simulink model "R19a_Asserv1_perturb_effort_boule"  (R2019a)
settings: Solver=ode15s  StartTime=0.0  StopTime=1  RelTol=1e-3  EnableMultiTasking=on
undefined symbols (not defined in the file): deg, kg, m, manette1_Défaut_sldprt, manette2_Défaut_sldprt, mm, N, rad, s, sigbuilder_block, STL, X, Y, Z
libraries: sm_lib x460, fl_lib x45, nesl_utility x23, simulink x3
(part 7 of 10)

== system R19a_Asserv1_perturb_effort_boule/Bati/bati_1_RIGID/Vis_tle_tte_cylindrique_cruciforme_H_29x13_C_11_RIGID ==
  ReferenceFrame : sm_lib/Frames and Transforms/Reference Frame
  Solid : sm_lib/Body Elements/Solid  InertiaType=Custom  Mass=8.3821869835456372e-05  MassUnits=kg  CenterOfMass=[4.9478681581074904 0.00064910481891303923 -0.0013634218224953438]  CenterOfMassUnits=mm  MomentsOfInertia=[0.00016543197172893975 0.0014334630955093895 0.0014333390308476422]  MomentsOfInertiaUnits=kg*mm^2  ProductsOfInertia=[-5.4062904633677868e-09 -1.3111174919527308e-07 6.0713893531177014e-07]  ProductsOfInertiaUnits=kg*mm^2  BasedOnType=Density  Density=1000  DensityUnits=kg/(m^3)  DoExposeReferenceFrame=on  SerializedFrames=<Frames/>  GraphicType=FromGeometry  MarkerShape=Sphere  MarkerSize=10  MarkerSizeUnits=m  GraphicVisPropType=SimpleVisualProperties  GraphicDiffuseColor=[0.75294117647058822 0.75294117647058822 0.75294117647058822]  GraphicSpecularColor=[0.5 0.5 0.5 1.0]  GraphicAmbientColor=[0.15 0.15 0.15 1.0]  GraphicEmissiveColor=[0.0 0.0 0.0 1.0]  GraphicShininess=75  GraphicOpacity=1  GeometryShape=FromFile  RectangleSize=[1 1]  RectangleSizeUnits=m  BrickDimensions=[1 1 1]  BrickDimensionUnits=m  CylinderRadius=1  CylinderRadiusUnits=m  CylinderLength=1  CylinderLengthUnits=m  SphereRadius=1  SphereRadiusUnits=m  EllipsoidRadii=[1 1 1]  EllipsoidRadiiUnits=m  ExtrusionCrossSection=[1 1; -1 1; -1 -1; 1 -1]  ExtrusionCrossSectionUnits=m  ExtrusionLength=1  ExtrusionLengthUnits=m  PolygonNumSides=3  PolygonOuterRadius=1  PolygonOuterRadiusUnits=m  ExtGeomFileType=STL  ExtGeomFileName=\STL\Vis à tôle tête cylindrique cruciforme H 2-9x13 - C_Réaliste_sldprt.STL  ExtGeomFileUnits=mm  RevolutionCrossSection=[1 1; 1 -1; 2 -1; 2 1]  RevolutionCrossSectionUnits=m  RevolutionExtent=Full  RevolutionAngle=180  RevolutionAngleUnits=deg
  F : PMIOPort  Side=Left
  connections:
  Solid/RConn1 -- ReferenceFrame/RConn1 -- F/RConn1

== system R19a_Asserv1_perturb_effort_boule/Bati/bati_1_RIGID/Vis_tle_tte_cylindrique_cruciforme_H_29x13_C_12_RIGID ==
  ReferenceFrame : sm_lib/Frames and Transforms/Reference Frame
  Solid : sm_lib/Body Elements/Solid  InertiaType=Custom  Mass=8.3821869835456372e-05  MassUnits=kg  CenterOfMass=[4.9478681581074904 0.00064910481891303923 -0.0013634218224953438]  CenterOfMassUnits=mm  MomentsOfInertia=[0.00016543197172893975 0.0014334630955093895 0.0014333390308476422]  MomentsOfInertiaUnits=kg*mm^2  ProductsOfInertia=[-5.4062904633677868e-09 -1.3111174919527308e-07 6.0713893531177014e-07]  ProductsOfInertiaUnits=kg*mm^2  BasedOnType=Density  Density=1000  DensityUnits=kg/(m^3)  DoExposeReferenceFrame=on  SerializedFrames=<Frames/>  GraphicType=FromGeometry  MarkerShape=Sphere  MarkerSize=10  MarkerSizeUnits=m  GraphicVisPropType=SimpleVisualProperties  GraphicDiffuseColor=[0.75294117647058822 0.75294117647058822 0.75294117647058822]  GraphicSpecularColor=[0.5 0.5 0.5 1.0]  GraphicAmbientColor=[0.15 0.15 0.15 1.0]  GraphicEmissiveColor=[0.0 0.0 0.0 1.0]  GraphicShininess=75  GraphicOpacity=1  GeometryShape=FromFile  RectangleSize=[1 1]  RectangleSizeUnits=m  BrickDimensions=[1 1 1]  BrickDimensionUnits=m  CylinderRadius=1  CylinderRadiusUnits=m  CylinderLength=1  CylinderLengthUnits=m  SphereRadius=1  SphereRadiusUnits=m  EllipsoidRadii=[1 1 1]  EllipsoidRadiiUnits=m  ExtrusionCrossSection=[1 1; -1 1; -1 -1; 1 -1]  ExtrusionCrossSectionUnits=m  ExtrusionLength=1  ExtrusionLengthUnits=m  PolygonNumSides=3  PolygonOuterRadius=1  PolygonOuterRadiusUnits=m  ExtGeomFileType=STL  ExtGeomFileName=\STL\Vis à tôle tête cylindrique cruciforme H 2-9x13 - C_Réaliste_sldprt.STL  ExtGeomFileUnits=mm  RevolutionCrossSection=[1 1; 1 -1; 2 -1; 2 1]  RevolutionCrossSectionUnits=m  RevolutionExtent=Full  RevolutionAngle=180  RevolutionAngleUnits=deg
  F : PMIOPort  Side=Left
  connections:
  Solid/RConn1 -- ReferenceFrame/RConn1 -- F/RConn1

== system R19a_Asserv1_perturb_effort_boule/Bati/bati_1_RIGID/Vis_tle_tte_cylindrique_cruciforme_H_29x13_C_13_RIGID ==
  ReferenceFrame : sm_lib/Frames and Transforms/Reference Frame
  Solid : sm_lib/Body Elements/Solid  InertiaType=Custom  Mass=8.3821869835456372e-05  MassUnits=kg  CenterOfMass=[4.9478681581074904 0.00064910481891303923 -0.0013634218224953438]  CenterOfMassUnits=mm  MomentsOfInertia=[0.00016543197172893975 0.0014334630955093895 0.0014333390308476422]  MomentsOfInertiaUnits=kg*mm^2  ProductsOfInertia=[-5.4062904633677868e-09 -1.3111174919527308e-07 6.0713893531177014e-07]  ProductsOfInertiaUnits=kg*mm^2  BasedOnType=Density  Density=1000  DensityUnits=kg/(m^3)  DoExposeReferenceFrame=on  SerializedFrames=<Frames/>  GraphicType=FromGeometry  MarkerShape=Sphere  MarkerSize=10  MarkerSizeUnits=m  GraphicVisPropType=SimpleVisualProperties  GraphicDiffuseColor=[0.75294117647058822 0.75294117647058822 0.75294117647058822]  GraphicSpecularColor=[0.5 0.5 0.5 1.0]  GraphicAmbientColor=[0.15 0.15 0.15 1.0]  GraphicEmissiveColor=[0.0 0.0 0.0 1.0]  GraphicShininess=75  GraphicOpacity=1  GeometryShape=FromFile  RectangleSize=[1 1]  RectangleSizeUnits=m  BrickDimensions=[1 1 1]  BrickDimensionUnits=m  CylinderRadius=1  CylinderRadiusUnits=m  CylinderLength=1  CylinderLengthUnits=m  SphereRadius=1  SphereRadiusUnits=m  EllipsoidRadii=[1 1 1]  EllipsoidRadiiUnits=m  ExtrusionCrossSection=[1 1; -1 1; -1 -1; 1 -1]  ExtrusionCrossSectionUnits=m  ExtrusionLength=1  ExtrusionLengthUnits=m  PolygonNumSides=3  PolygonOuterRadius=1  PolygonOuterRadiusUnits=m  ExtGeomFileType=STL  ExtGeomFileName=\STL\Vis à tôle tête cylindrique cruciforme H 2-9x13 - C_Réaliste_sldprt.STL  ExtGeomFileUnits=mm  RevolutionCrossSection=[1 1; 1 -1; 2 -1; 2 1]  RevolutionCrossSectionUnits=m  RevolutionExtent=Full  RevolutionAngle=180  RevolutionAngleUnits=deg
  F : PMIOPort  Side=Left
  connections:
  Solid/RConn1 -- ReferenceFrame/RConn1 -- F/RConn1

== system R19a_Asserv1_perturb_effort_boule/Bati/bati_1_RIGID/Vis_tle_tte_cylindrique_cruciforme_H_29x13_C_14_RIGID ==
  ReferenceFrame : sm_lib/Frames and Transforms/Reference Frame
  Solid : sm_lib/Body Elements/Solid  InertiaType=Custom  Mass=8.3821869835456372e-05  MassUnits=kg  CenterOfMass=[4.9478681581074904 0.00064910481891303923 -0.0013634218224953438]  CenterOfMassUnits=mm  MomentsOfInertia=[0.00016543197172893975 0.0014334630955093895 0.0014333390308476422]  MomentsOfInertiaUnits=kg*mm^2  ProductsOfInertia=[-5.4062904633677868e-09 -1.3111174919527308e-07 6.0713893531177014e-07]  ProductsOfInertiaUnits=kg*mm^2  BasedOnType=Density  Density=1000  DensityUnits=kg/(m^3)  DoExposeReferenceFrame=on  SerializedFrames=<Frames/>  GraphicType=FromGeometry  MarkerShape=Sphere  MarkerSize=10  MarkerSizeUnits=m  GraphicVisPropType=SimpleVisualProperties  GraphicDiffuseColor=[0.75294117647058822 0.75294117647058822 0.75294117647058822]  GraphicSpecularColor=[0.5 0.5 0.5 1.0]  GraphicAmbientColor=[0.15 0.15 0.15 1.0]  GraphicEmissiveColor=[0.0 0.0 0.0 1.0]  GraphicShininess=75  GraphicOpacity=1  GeometryShape=FromFile  RectangleSize=[1 1]  RectangleSizeUnits=m  BrickDimensions=[1 1 1]  BrickDimensionUnits=m  CylinderRadius=1  CylinderRadiusUnits=m  CylinderLength=1  CylinderLengthUnits=m  SphereRadius=1  SphereRadiusUnits=m  EllipsoidRadii=[1 1 1]  EllipsoidRadiiUnits=m  ExtrusionCrossSection=[1 1; -1 1; -1 -1; 1 -1]  ExtrusionCrossSectionUnits=m  ExtrusionLength=1  ExtrusionLengthUnits=m  PolygonNumSides=3  PolygonOuterRadius=1  PolygonOuterRadiusUnits=m  ExtGeomFileType=STL  ExtGeomFileName=\STL\Vis à tôle tête cylindrique cruciforme H 2-9x13 - C_Réaliste_sldprt.STL  ExtGeomFileUnits=mm  RevolutionCrossSection=[1 1; 1 -1; 2 -1; 2 1]  RevolutionCrossSectionUnits=m  RevolutionExtent=Full  RevolutionAngle=180  RevolutionAngleUnits=deg
  F : PMIOPort  Side=Left
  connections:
  Solid/RConn1 -- ReferenceFrame/RConn1 -- F/RConn1

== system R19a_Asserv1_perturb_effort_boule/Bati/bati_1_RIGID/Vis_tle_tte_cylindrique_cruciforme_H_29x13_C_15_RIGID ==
  ReferenceFrame : sm_lib/Frames and Transforms/Reference Frame
  Solid : sm_lib/Body Elements/Solid  InertiaType=Custom  Mass=8.3821869835456372e-05  MassUnits=kg  CenterOfMass=[4.9478681581074904 0.00064910481891303923 -0.0013634218224953438]  CenterOfMassUnits=mm  MomentsOfInertia=[0.00016543197172893975 0.0014334630955093895 0.0014333390308476422]  MomentsOfInertiaUnits=kg*mm^2  ProductsOfInertia=[-5.4062904633677868e-09 -1.3111174919527308e-07 6.0713893531177014e-07]  ProductsOfInertiaUnits=kg*mm^2  BasedOnType=Density  Density=1000  DensityUnits=kg/(m^3)  DoExposeReferenceFrame=on  SerializedFrames=<Frames/>  GraphicType=FromGeometry  MarkerShape=Sphere  MarkerSize=10  MarkerSizeUnits=m  GraphicVisPropType=SimpleVisualProperties  GraphicDiffuseColor=[0.75294117647058822 0.75294117647058822 0.75294117647058822]  GraphicSpecularColor=[0.5 0.5 0.5 1.0]  GraphicAmbientColor=[0.15 0.15 0.15 1.0]  GraphicEmissiveColor=[0.0 0.0 0.0 1.0]  GraphicShininess=75  GraphicOpacity=1  GeometryShape=FromFile  RectangleSize=[1 1]  RectangleSizeUnits=m  BrickDimensions=[1 1 1]  BrickDimensionUnits=m  CylinderRadius=1  CylinderRadiusUnits=m  CylinderLength=1  CylinderLengthUnits=m  SphereRadius=1  SphereRadiusUnits=m  EllipsoidRadii=[1 1 1]  EllipsoidRadiiUnits=m  ExtrusionCrossSection=[1 1; -1 1; -1 -1; 1 -1]  ExtrusionCrossSectionUnits=m  ExtrusionLength=1  ExtrusionLengthUnits=m  PolygonNumSides=3  PolygonOuterRadius=1  PolygonOuterRadiusUnits=m  ExtGeomFileType=STL  ExtGeomFileName=\STL\Vis à tôle tête cylindrique cruciforme H 2-9x13 - C_Réaliste_sldprt.STL  ExtGeomFileUnits=mm  RevolutionCrossSection=[1 1; 1 -1; 2 -1; 2 1]  RevolutionCrossSectionUnits=m  RevolutionExtent=Full  RevolutionAngle=180  RevolutionAngleUnits=deg
  F : PMIOPort  Side=Left
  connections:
  Solid/RConn1 -- ReferenceFrame/RConn1 -- F/RConn1

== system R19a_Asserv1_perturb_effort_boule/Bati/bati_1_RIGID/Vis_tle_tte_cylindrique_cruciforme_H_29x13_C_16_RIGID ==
  ReferenceFrame : sm_lib/Frames and Transforms/Reference Frame
  Solid : sm_lib/Body Elements/Solid  InertiaType=Custom  Mass=8.3821869835456372e-05  MassUnits=kg  CenterOfMass=[4.9478681581074904 0.00064910481891303923 -0.0013634218224953438]  CenterOfMassUnits=mm  MomentsOfInertia=[0.00016543197172893975 0.0014334630955093895 0.0014333390308476422]  MomentsOfInertiaUnits=kg*mm^2  ProductsOfInertia=[-5.4062904633677868e-09 -1.3111174919527308e-07 6.0713893531177014e-07]  ProductsOfInertiaUnits=kg*mm^2  BasedOnType=Density  Density=1000  DensityUnits=kg/(m^3)  DoExposeReferenceFrame=on  SerializedFrames=<Frames/>  GraphicType=FromGeometry  MarkerShape=Sphere  MarkerSize=10  MarkerSizeUnits=m  GraphicVisPropType=SimpleVisualProperties  GraphicDiffuseColor=[0.75294117647058822 0.75294117647058822 0.75294117647058822]  GraphicSpecularColor=[0.5 0.5 0.5 1.0]  GraphicAmbientColor=[0.15 0.15 0.15 1.0]  GraphicEmissiveColor=[0.0 0.0 0.0 1.0]  GraphicShininess=75  GraphicOpacity=1  GeometryShape=FromFile  RectangleSize=[1 1]  RectangleSizeUnits=m  BrickDimensions=[1 1 1]  BrickDimensionUnits=m  CylinderRadius=1  CylinderRadiusUnits=m  CylinderLength=1  CylinderLengthUnits=m  SphereRadius=1  SphereRadiusUnits=m  EllipsoidRadii=[1 1 1]  EllipsoidRadiiUnits=m  ExtrusionCrossSection=[1 1; -1 1; -1 -1; 1 -1]  ExtrusionCrossSectionUnits=m  ExtrusionLength=1  ExtrusionLengthUnits=m  PolygonNumSides=3  PolygonOuterRadius=1  PolygonOuterRadiusUnits=m  ExtGeomFileType=STL  ExtGeomFileName=\STL\Vis à tôle tête cylindrique cruciforme H 2-9x13 - C_Réaliste_sldprt.STL  ExtGeomFileUnits=mm  RevolutionCrossSection=[1 1; 1 -1; 2 -1; 2 1]  RevolutionCrossSectionUnits=m  RevolutionExtent=Full  RevolutionAngle=180  RevolutionAngleUnits=deg
  F : PMIOPort  Side=Left
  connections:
  Solid/RConn1 -- ReferenceFrame/RConn1 -- F/RConn1

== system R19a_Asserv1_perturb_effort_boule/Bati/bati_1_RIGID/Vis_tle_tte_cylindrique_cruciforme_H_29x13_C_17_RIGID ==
  ReferenceFrame : sm_lib/Frames and Transforms/Reference Frame
  Solid : sm_lib/Body Elements/Solid  InertiaType=Custom  Mass=8.3821869835456372e-05  MassUnits=kg  CenterOfMass=[4.9478681581074904 0.00064910481891303923 -0.0013634218224953438]  CenterOfMassUnits=mm  MomentsOfInertia=[0.00016543197172893975 0.0014334630955093895 0.0014333390308476422]  MomentsOfInertiaUnits=kg*mm^2  ProductsOfInertia=[-5.4062904633677868e-09 -1.3111174919527308e-07 6.0713893531177014e-07]  ProductsOfInertiaUnits=kg*mm^2  BasedOnType=Density  Density=1000  DensityUnits=kg/(m^3)  DoExposeReferenceFrame=on  SerializedFrames=<Frames/>  GraphicType=FromGeometry  MarkerShape=Sphere  MarkerSize=10  MarkerSizeUnits=m  GraphicVisPropType=SimpleVisualProperties  GraphicDiffuseColor=[0.75294117647058822 0.75294117647058822 0.75294117647058822]  GraphicSpecularColor=[0.5 0.5 0.5 1.0]  GraphicAmbientColor=[0.15 0.15 0.15 1.0]  GraphicEmissiveColor=[0.0 0.0 0.0 1.0]  GraphicShininess=75  GraphicOpacity=1  GeometryShape=FromFile  RectangleSize=[1 1]  RectangleSizeUnits=m  BrickDimensions=[1 1 1]  BrickDimensionUnits=m  CylinderRadius=1  CylinderRadiusUnits=m  CylinderLength=1  CylinderLengthUnits=m  SphereRadius=1  SphereRadiusUnits=m  EllipsoidRadii=[1 1 1]  EllipsoidRadiiUnits=m  ExtrusionCrossSection=[1 1; -1 1; -1 -1; 1 -1]  ExtrusionCrossSectionUnits=m  ExtrusionLength=1  ExtrusionLengthUnits=m  PolygonNumSides=3  PolygonOuterRadius=1  PolygonOuterRadiusUnits=m  ExtGeomFileType=STL  ExtGeomFileName=\STL\Vis à tôle tête cylindrique cruciforme H 2-9x13 - C_Réaliste_sldprt.STL  ExtGeomFileUnits=mm  RevolutionCrossSection=[1 1; 1 -1; 2 -1; 2 1]  RevolutionCrossSectionUnits=m  RevolutionExtent=Full  RevolutionAngle=180  RevolutionAngleUnits=deg
  F : PMIOPort  Side=Left
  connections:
  Solid/RConn1 -- ReferenceFrame/RConn1 -- F/RConn1

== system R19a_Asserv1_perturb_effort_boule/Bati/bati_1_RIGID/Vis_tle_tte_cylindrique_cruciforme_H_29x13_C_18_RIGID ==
  ReferenceFrame : sm_lib/Frames and Transforms/Reference Frame
  Solid : sm_lib/Body Elements/Solid  InertiaType=Custom  Mass=8.3821869835456372e-05  MassUnits=kg  CenterOfMass=[4.9478681581074904 0.00064910481891303923 -0.0013634218224953438]  CenterOfMassUnits=mm  MomentsOfInertia=[0.00016543197172893975 0.0014334630955093895 0.0014333390308476422]  MomentsOfInertiaUnits=kg*mm^2  ProductsOfInertia=[-5.4062904633677868e-09 -1.3111174919527308e-07 6.0713893531177014e-07]  ProductsOfInertiaUnits=kg*mm^2  BasedOnType=Density  Density=1000  DensityUnits=kg/(m^3)  DoExposeReferenceFrame=on  SerializedFrames=<Frames/>  GraphicType=FromGeometry  MarkerShape=Sphere  MarkerSize=10  MarkerSizeUnits=m  GraphicVisPropType=SimpleVisualProperties  GraphicDiffuseColor=[0.75294117647058822 0.75294117647058822 0.75294117647058822]  GraphicSpecularColor=[0.5 0.5 0.5 1.0]  GraphicAmbientColor=[0.15 0.15 0.15 1.0]  GraphicEmissiveColor=[0.0 0.0 0.0 1.0]  GraphicShininess=75  GraphicOpacity=1  GeometryShape=FromFile  RectangleSize=[1 1]  RectangleSizeUnits=m  BrickDimensions=[1 1 1]  BrickDimensionUnits=m  CylinderRadius=1  CylinderRadiusUnits=m  CylinderLength=1  CylinderLengthUnits=m  SphereRadius=1  SphereRadiusUnits=m  EllipsoidRadii=[1 1 1]  EllipsoidRadiiUnits=m  ExtrusionCrossSection=[1 1; -1 1; -1 -1; 1 -1]  ExtrusionCrossSectionUnits=m  ExtrusionLength=1  ExtrusionLengthUnits=m  PolygonNumSides=3  PolygonOuterRadius=1  PolygonOuterRadiusUnits=m  ExtGeomFileType=STL  ExtGeomFileName=\STL\Vis à tôle tête cylindrique cruciforme H 2-9x13 - C_Réaliste_sldprt.STL  ExtGeomFileUnits=mm  RevolutionCrossSection=[1 1; 1 -1; 2 -1; 2 1]  RevolutionCrossSectionUnits=m  RevolutionExtent=Full  RevolutionAngle=180  RevolutionAngleUnits=deg
  F : PMIOPort  Side=Left
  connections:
  Solid/RConn1 -- ReferenceFrame/RConn1 -- F/RConn1

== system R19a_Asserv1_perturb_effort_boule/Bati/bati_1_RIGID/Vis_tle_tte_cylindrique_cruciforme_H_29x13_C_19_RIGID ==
  ReferenceFrame : sm_lib/Frames and Transforms/Reference Frame
  Solid : sm_lib/Body Elements/Solid  InertiaType=Custom  Mass=8.3821869835456372e-05  MassUnits=kg  CenterOfMass=[4.9478681581074904 0.00064910481891303923 -0.0013634218224953438]  CenterOfMassUnits=mm  MomentsOfInertia=[0.00016543197172893975 0.0014334630955093895 0.0014333390308476422]  MomentsOfInertiaUnits=kg*mm^2  ProductsOfInertia=[-5.4062904633677868e-09 -1.3111174919527308e-07 6.0713893531177014e-07]  ProductsOfInertiaUnits=kg*mm^2  BasedOnType=Density  Density=1000  DensityUnits=kg/(m^3)  DoExposeReferenceFrame=on  SerializedFrames=<Frames/>  GraphicType=FromGeometry  MarkerShape=Sphere  MarkerSize=10  MarkerSizeUnits=m  GraphicVisPropType=SimpleVisualProperties  GraphicDiffuseColor=[0.75294117647058822 0.75294117647058822 0.75294117647058822]  GraphicSpecularColor=[0.5 0.5 0.5 1.0]  GraphicAmbientColor=[0.15 0.15 0.15 1.0]  GraphicEmissiveColor=[0.0 0.0 0.0 1.0]  GraphicShininess=75  GraphicOpacity=1  GeometryShape=FromFile  RectangleSize=[1 1]  RectangleSizeUnits=m  BrickDimensions=[1 1 1]  BrickDimensionUnits=m  CylinderRadius=1  CylinderRadiusUnits=m  CylinderLength=1  CylinderLengthUnits=m  SphereRadius=1  SphereRadiusUnits=m  EllipsoidRadii=[1 1 1]  EllipsoidRadiiUnits=m  ExtrusionCrossSection=[1 1; -1 1; -1 -1; 1 -1]  ExtrusionCrossSectionUnits=m  ExtrusionLength=1  ExtrusionLengthUnits=m  PolygonNumSides=3  PolygonOuterRadius=1  PolygonOuterRadiusUnits=m  ExtGeomFileType=STL  ExtGeomFileName=\STL\Vis à tôle tête cylindrique cruciforme H 2-9x13 - C_Réaliste_sldprt.STL  ExtGeomFileUnits=mm  RevolutionCrossSection=[1 1; 1 -1; 2 -1; 2 1]  RevolutionCrossSectionUnits=m  RevolutionExtent=Full  RevolutionAngle=180  RevolutionAngleUnits=deg
  F : PMIOPort  Side=Left
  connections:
  Solid/RConn1 -- ReferenceFrame/RConn1 -- F/RConn1

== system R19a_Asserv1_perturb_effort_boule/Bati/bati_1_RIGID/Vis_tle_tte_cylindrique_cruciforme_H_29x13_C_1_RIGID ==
  ReferenceFrame : sm_lib/Frames and Transforms/Reference Frame
  Solid : sm_lib/Body Elements/Solid  InertiaType=Custom  Mass=8.3821869835456372e-05  MassUnits=kg  CenterOfMass=[4.9478681581074904 0.00064910481891303923 -0.0013634218224953438]  CenterOfMassUnits=mm  MomentsOfInertia=[0.00016543197172893975 0.0014334630955093895 0.0014333390308476422]  MomentsOfInertiaUnits=kg*mm^2  ProductsOfInertia=[-5.4062904633677868e-09 -1.3111174919527308e-07 6.0713893531177014e-07]  ProductsOfInertiaUnits=kg*mm^2  BasedOnType=Density  Density=1000  DensityUnits=kg/(m^3)  DoExposeReferenceFrame=on  SerializedFrames=<Frames/>  GraphicType=FromGeometry  MarkerShape=Sphere  MarkerSize=10  MarkerSizeUnits=m  GraphicVisPropType=SimpleVisualProperties  GraphicDiffuseColor=[0.75294117647058822 0.75294117647058822 0.75294117647058822]  GraphicSpecularColor=[0.5 0.5 0.5 1.0]  GraphicAmbientColor=[0.15 0.15 0.15 1.0]  GraphicEmissiveColor=[0.0 0.0 0.0 1.0]  GraphicShininess=75  GraphicOpacity=1  GeometryShape=FromFile  RectangleSize=[1 1]  RectangleSizeUnits=m  BrickDimensions=[1 1 1]  BrickDimensionUnits=m  CylinderRadius=1  CylinderRadiusUnits=m  CylinderLength=1  CylinderLengthUnits=m  SphereRadius=1  SphereRadiusUnits=m  EllipsoidRadii=[1 1 1]  EllipsoidRadiiUnits=m  ExtrusionCrossSection=[1 1; -1 1; -1 -1; 1 -1]  ExtrusionCrossSectionUnits=m  ExtrusionLength=1  ExtrusionLengthUnits=m  PolygonNumSides=3  PolygonOuterRadius=1  PolygonOuterRadiusUnits=m  ExtGeomFileType=STL  ExtGeomFileName=\STL\Vis à tôle tête cylindrique cruciforme H 2-9x13 - C_Réaliste_sldprt.STL  ExtGeomFileUnits=mm  RevolutionCrossSection=[1 1; 1 -1; 2 -1; 2 1]  RevolutionCrossSectionUnits=m  RevolutionExtent=Full  RevolutionAngle=180  RevolutionAngleUnits=deg
  F : PMIOPort  Side=Left
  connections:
  Solid/RConn1 -- ReferenceFrame/RConn1 -- F/RConn1

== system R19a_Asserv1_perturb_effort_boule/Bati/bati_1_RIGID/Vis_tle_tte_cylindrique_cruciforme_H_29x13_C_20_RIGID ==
  ReferenceFrame : sm_lib/Frames and Transforms/Reference Frame
  Solid : sm_lib/Body Elements/Solid  InertiaType=Custom  Mass=8.3821869835456372e-05  MassUnits=kg  CenterOfMass=[4.9478681581074904 0.00064910481891303923 -0.0013634218224953438]  CenterOfMassUnits=mm  MomentsOfInertia=[0.00016543197172893975 0.0014334630955093895 0.0014333390308476422]  MomentsOfInertiaUnits=kg*mm^2  ProductsOfInertia=[-5.4062904633677868e-09 -1.3111174919527308e-07 6.0713893531177014e-07]  ProductsOfInertiaUnits=kg*mm^2  BasedOnType=Density  Density=1000  DensityUnits=kg/(m^3)  DoExposeReferenceFrame=on  SerializedFrames=<Frames/>  GraphicType=FromGeometry  MarkerShape=Sphere  MarkerSize=10  MarkerSizeUnits=m  GraphicVisPropType=SimpleVisualProperties  GraphicDiffuseColor=[0.75294117647058822 0.75294117647058822 0.75294117647058822]  GraphicSpecularColor=[0.5 0.5 0.5 1.0]  GraphicAmbientColor=[0.15 0.15 0.15 1.0]  GraphicEmissiveColor=[0.0 0.0 0.0 1.0]  GraphicShininess=75  GraphicOpacity=1  GeometryShape=FromFile  RectangleSize=[1 1]  RectangleSizeUnits=m  BrickDimensions=[1 1 1]  BrickDimensionUnits=m  CylinderRadius=1  CylinderRadiusUnits=m  CylinderLength=1  CylinderLengthUnits=m  SphereRadius=1  SphereRadiusUnits=m  EllipsoidRadii=[1 1 1]  EllipsoidRadiiUnits=m  ExtrusionCrossSection=[1 1; -1 1; -1 -1; 1 -1]  ExtrusionCrossSectionUnits=m  ExtrusionLength=1  ExtrusionLengthUnits=m  PolygonNumSides=3  PolygonOuterRadius=1  PolygonOuterRadiusUnits=m  ExtGeomFileType=STL  ExtGeomFileName=\STL\Vis à tôle tête cylindrique cruciforme H 2-9x13 - C_Réaliste_sldprt.STL  ExtGeomFileUnits=mm  RevolutionCrossSection=[1 1; 1 -1; 2 -1; 2 1]  RevolutionCrossSectionUnits=m  RevolutionExtent=Full  RevolutionAngle=180  RevolutionAngleUnits=deg
  F : PMIOPort  Side=Left
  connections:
  Solid/RConn1 -- ReferenceFrame/RConn1 -- F/RConn1

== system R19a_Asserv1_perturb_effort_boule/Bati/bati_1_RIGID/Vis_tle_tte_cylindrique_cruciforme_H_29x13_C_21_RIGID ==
  ReferenceFrame : sm_lib/Frames and Transforms/Reference Frame
  Solid : sm_lib/Body Elements/Solid  InertiaType=Custom  Mass=8.3821869835456372e-05  MassUnits=kg  CenterOfMass=[4.9478681581074904 0.00064910481891303923 -0.0013634218224953438]  CenterOfMassUnits=mm  MomentsOfInertia=[0.00016543197172893975 0.0014334630955093895 0.0014333390308476422]  MomentsOfInertiaUnits=kg*mm^2  ProductsOfInertia=[-5.4062904633677868e-09 -1.3111174919527308e-07 6.0713893531177014e-07]  ProductsOfInertiaUnits=kg*mm^2  BasedOnType=Density  Density=1000  DensityUnits=kg/(m^3)  DoExposeReferenceFrame=on  SerializedFrames=<Frames/>  GraphicType=FromGeometry  MarkerShape=Sphere  MarkerSize=10  MarkerSizeUnits=m  GraphicVisPropType=SimpleVisualProperties  GraphicDiffuseColor=[0.75294117647058822 0.75294117647058822 0.75294117647058822]  GraphicSpecularColor=[0.5 0.5 0.5 1.0]  GraphicAmbientColor=[0.15 0.15 0.15 1.0]  GraphicEmissiveColor=[0.0 0.0 0.0 1.0]  GraphicShininess=75  GraphicOpacity=1  GeometryShape=FromFile  RectangleSize=[1 1]  RectangleSizeUnits=m  BrickDimensions=[1 1 1]  BrickDimensionUnits=m  CylinderRadius=1  CylinderRadiusUnits=m  CylinderLength=1  CylinderLengthUnits=m  SphereRadius=1  SphereRadiusUnits=m  EllipsoidRadii=[1 1 1]  EllipsoidRadiiUnits=m  ExtrusionCrossSection=[1 1; -1 1; -1 -1; 1 -1]  ExtrusionCrossSectionUnits=m  ExtrusionLength=1  ExtrusionLengthUnits=m  PolygonNumSides=3  PolygonOuterRadius=1  PolygonOuterRadiusUnits=m  ExtGeomFileType=STL  ExtGeomFileName=\STL\Vis à tôle tête cylindrique cruciforme H 2-9x13 - C_Réaliste_sldprt.STL  ExtGeomFileUnits=mm  RevolutionCrossSection=[1 1; 1 -1; 2 -1; 2 1]  RevolutionCrossSectionUnits=m  RevolutionExtent=Full  RevolutionAngle=180  RevolutionAngleUnits=deg
  F : PMIOPort  Side=Left
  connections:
  Solid/RConn1 -- ReferenceFrame/RConn1 -- F/RConn1

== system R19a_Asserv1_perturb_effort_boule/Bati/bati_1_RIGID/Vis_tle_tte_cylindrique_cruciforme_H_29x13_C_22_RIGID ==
  ReferenceFrame : sm_lib/Frames and Transforms/Reference Frame
  Solid : sm_lib/Body Elements/Solid  InertiaType=Custom  Mass=8.3821869835456372e-05  MassUnits=kg  CenterOfMass=[4.9478681581074904 0.00064910481891303923 -0.0013634218224953438]  CenterOfMassUnits=mm  MomentsOfInertia=[0.00016543197172893975 0.0014334630955093895 0.0014333390308476422]  MomentsOfInertiaUnits=kg*mm^2  ProductsOfInertia=[-5.4062904633677868e-09 -1.3111174919527308e-07 6.0713893531177014e-07]  ProductsOfInertiaUnits=kg*mm^2  BasedOnType=Density  Density=1000  DensityUnits=kg/(m^3)  DoExposeReferenceFrame=on  SerializedFrames=<Frames/>  GraphicType=FromGeometry  MarkerShape=Sphere  MarkerSize=10  MarkerSizeUnits=m  GraphicVisPropType=SimpleVisualProperties  GraphicDiffuseColor=[0.75294117647058822 0.75294117647058822 0.75294117647058822]  GraphicSpecularColor=[0.5 0.5 0.5 1.0]  GraphicAmbientColor=[0.15 0.15 0.15 1.0]  GraphicEmissiveColor=[0.0 0.0 0.0 1.0]  GraphicShininess=75  GraphicOpacity=1  GeometryShape=FromFile  RectangleSize=[1 1]  RectangleSizeUnits=m  BrickDimensions=[1 1 1]  BrickDimensionUnits=m  CylinderRadius=1  CylinderRadiusUnits=m  CylinderLength=1  CylinderLengthUnits=m  SphereRadius=1  SphereRadiusUnits=m  EllipsoidRadii=[1 1 1]  EllipsoidRadiiUnits=m  ExtrusionCrossSection=[1 1; -1 1; -1 -1; 1 -1]  ExtrusionCrossSectionUnits=m  ExtrusionLength=1  ExtrusionLengthUnits=m  PolygonNumSides=3  PolygonOuterRadius=1  PolygonOuterRadiusUnits=m  ExtGeomFileType=STL  ExtGeomFileName=\STL\Vis à tôle tête cylindrique cruciforme H 2-9x13 - C_Réaliste_sldprt.STL  ExtGeomFileUnits=mm  RevolutionCrossSection=[1 1; 1 -1; 2 -1; 2 1]  RevolutionCrossSectionUnits=m  RevolutionExtent=Full  RevolutionAngle=180  RevolutionAngleUnits=deg
  F : PMIOPort  Side=Left
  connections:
  Solid/RConn1 -- ReferenceFrame/RConn1 -- F/RConn1

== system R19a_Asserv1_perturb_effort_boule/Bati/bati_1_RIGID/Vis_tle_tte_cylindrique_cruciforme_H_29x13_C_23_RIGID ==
  ReferenceFrame : sm_lib/Frames and Transforms/Reference Frame
  Solid : sm_lib/Body Elements/Solid  InertiaType=Custom  Mass=8.3821869835456372e-05  MassUnits=kg  CenterOfMass=[4.9478681581074904 0.00064910481891303923 -0.0013634218224953438]  CenterOfMassUnits=mm  MomentsOfInertia=[0.00016543197172893975 0.0014334630955093895 0.0014333390308476422]  MomentsOfInertiaUnits=kg*mm^2  ProductsOfInertia=[-5.4062904633677868e-09 -1.3111174919527308e-07 6.0713893531177014e-07]  ProductsOfInertiaUnits=kg*mm^2  BasedOnType=Density  Density=1000  DensityUnits=kg/(m^3)  DoExposeReferenceFrame=on  SerializedFrames=<Frames/>  GraphicType=FromGeometry  MarkerShape=Sphere  MarkerSize=10  MarkerSizeUnits=m  GraphicVisPropType=SimpleVisualProperties  GraphicDiffuseColor=[0.75294117647058822 0.75294117647058822 0.75294117647058822]  GraphicSpecularColor=[0.5 0.5 0.5 1.0]  GraphicAmbientColor=[0.15 0.15 0.15 1.0]  GraphicEmissiveColor=[0.0 0.0 0.0 1.0]  GraphicShininess=75  GraphicOpacity=1  GeometryShape=FromFile  RectangleSize=[1 1]  RectangleSizeUnits=m  BrickDimensions=[1 1 1]  BrickDimensionUnits=m  CylinderRadius=1  CylinderRadiusUnits=m  CylinderLength=1  CylinderLengthUnits=m  SphereRadius=1  SphereRadiusUnits=m  EllipsoidRadii=[1 1 1]  EllipsoidRadiiUnits=m  ExtrusionCrossSection=[1 1; -1 1; -1 -1; 1 -1]  ExtrusionCrossSectionUnits=m  ExtrusionLength=1  ExtrusionLengthUnits=m  PolygonNumSides=3  PolygonOuterRadius=1  PolygonOuterRadiusUnits=m  ExtGeomFileType=STL  ExtGeomFileName=\STL\Vis à tôle tête cylindrique cruciforme H 2-9x13 - C_Réaliste_sldprt.STL  ExtGeomFileUnits=mm  RevolutionCrossSection=[1 1; 1 -1; 2 -1; 2 1]  RevolutionCrossSectionUnits=m  RevolutionExtent=Full  RevolutionAngle=180  RevolutionAngleUnits=deg
  F : PMIOPort  Side=Left
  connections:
  Solid/RConn1 -- ReferenceFrame/RConn1 -- F/RConn1

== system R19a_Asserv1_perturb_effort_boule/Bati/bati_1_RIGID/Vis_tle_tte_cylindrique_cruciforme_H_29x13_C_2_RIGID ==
  ReferenceFrame : sm_lib/Frames and Transforms/Reference Frame
  Solid : sm_lib/Body Elements/Solid  InertiaType=Custom  Mass=8.3821869835456372e-05  MassUnits=kg  CenterOfMass=[4.9478681581074904 0.00064910481891303923 -0.0013634218224953438]  CenterOfMassUnits=mm  MomentsOfInertia=[0.00016543197172893975 0.0014334630955093895 0.0014333390308476422]  MomentsOfInertiaUnits=kg*mm^2  ProductsOfInertia=[-5.4062904633677868e-09 -1.3111174919527308e-07 6.0713893531177014e-07]  ProductsOfInertiaUnits=kg*mm^2  BasedOnType=Density  Density=1000  DensityUnits=kg/(m^3)  DoExposeReferenceFrame=on  SerializedFrames=<Frames/>  GraphicType=FromGeometry  MarkerShape=Sphere  MarkerSize=10  MarkerSizeUnits=m  GraphicVisPropType=SimpleVisualProperties  GraphicDiffuseColor=[0.75294117647058822 0.75294117647058822 0.75294117647058822]  GraphicSpecularColor=[0.5 0.5 0.5 1.0]  GraphicAmbientColor=[0.15 0.15 0.15 1.0]  GraphicEmissiveColor=[0.0 0.0 0.0 1.0]  GraphicShininess=75  GraphicOpacity=1  GeometryShape=FromFile  RectangleSize=[1 1]  RectangleSizeUnits=m  BrickDimensions=[1 1 1]  BrickDimensionUnits=m  CylinderRadius=1  CylinderRadiusUnits=m  CylinderLength=1  CylinderLengthUnits=m  SphereRadius=1  SphereRadiusUnits=m  EllipsoidRadii=[1 1 1]  EllipsoidRadiiUnits=m  ExtrusionCrossSection=[1 1; -1 1; -1 -1; 1 -1]  ExtrusionCrossSectionUnits=m  ExtrusionLength=1  ExtrusionLengthUnits=m  PolygonNumSides=3  PolygonOuterRadius=1  PolygonOuterRadiusUnits=m  ExtGeomFileType=STL  ExtGeomFileName=\STL\Vis à tôle tête cylindrique cruciforme H 2-9x13 - C_Réaliste_sldprt.STL  ExtGeomFileUnits=mm  RevolutionCrossSection=[1 1; 1 -1; 2 -1; 2 1]  RevolutionCrossSectionUnits=m  RevolutionExtent=Full  RevolutionAngle=180  RevolutionAngleUnits=deg
  F : PMIOPort  Side=Left
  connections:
  Solid/RConn1 -- ReferenceFrame/RConn1 -- F/RConn1

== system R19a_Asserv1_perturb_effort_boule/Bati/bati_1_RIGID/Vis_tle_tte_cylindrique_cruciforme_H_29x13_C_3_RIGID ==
  ReferenceFrame : sm_lib/Frames and Transforms/Reference Frame
  Solid : sm_lib/Body Elements/Solid  InertiaType=Custom  Mass=8.3821869835456372e-05  MassUnits=kg  CenterOfMass=[4.9478681581074904 0.00064910481891303923 -0.0013634218224953438]  CenterOfMassUnits=mm  MomentsOfInertia=[0.00016543197172893975 0.0014334630955093895 0.0014333390308476422]  MomentsOfInertiaUnits=kg*mm^2  ProductsOfInertia=[-5.4062904633677868e-09 -1.3111174919527308e-07 6.0713893531177014e-07]  ProductsOfInertiaUnits=kg*mm^2  BasedOnType=Density  Density=1000  DensityUnits=kg/(m^3)  DoExposeReferenceFrame=on  SerializedFrames=<Frames/>  GraphicType=FromGeometry  MarkerShape=Sphere  MarkerSize=10  MarkerSizeUnits=m  GraphicVisPropType=SimpleVisualProperties  GraphicDiffuseColor=[0.75294117647058822 0.75294117647058822 0.75294117647058822]  GraphicSpecularColor=[0.5 0.5 0.5 1.0]  GraphicAmbientColor=[0.15 0.15 0.15 1.0]  GraphicEmissiveColor=[0.0 0.0 0.0 1.0]  GraphicShininess=75  GraphicOpacity=1  GeometryShape=FromFile  RectangleSize=[1 1]  RectangleSizeUnits=m  BrickDimensions=[1 1 1]  BrickDimensionUnits=m  CylinderRadius=1  CylinderRadiusUnits=m  CylinderLength=1  CylinderLengthUnits=m  SphereRadius=1  SphereRadiusUnits=m  EllipsoidRadii=[1 1 1]  EllipsoidRadiiUnits=m  ExtrusionCrossSection=[1 1; -1 1; -1 -1; 1 -1]  ExtrusionCrossSectionUnits=m  ExtrusionLength=1  ExtrusionLengthUnits=m  PolygonNumSides=3  PolygonOuterRadius=1  PolygonOuterRadiusUnits=m  ExtGeomFileType=STL  ExtGeomFileName=\STL\Vis à tôle tête cylindrique cruciforme H 2-9x13 - C_Réaliste_sldprt.STL  ExtGeomFileUnits=mm  RevolutionCrossSection=[1 1; 1 -1; 2 -1; 2 1]  RevolutionCrossSectionUnits=m  RevolutionExtent=Full  RevolutionAngle=180  RevolutionAngleUnits=deg
  F : PMIOPort  Side=Left
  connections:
  Solid/RConn1 -- ReferenceFrame/RConn1 -- F/RConn1

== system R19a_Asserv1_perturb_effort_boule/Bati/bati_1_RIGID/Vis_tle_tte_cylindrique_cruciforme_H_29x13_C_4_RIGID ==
  ReferenceFrame : sm_lib/Frames and Transforms/Reference Frame
  Solid : sm_lib/Body Elements/Solid  InertiaType=Custom  Mass=8.3821869835456372e-05  MassUnits=kg  CenterOfMass=[4.9478681581074904 0.00064910481891303923 -0.0013634218224953438]  CenterOfMassUnits=mm  MomentsOfInertia=[0.00016543197172893975 0.0014334630955093895 0.0014333390308476422]  MomentsOfInertiaUnits=kg*mm^2  ProductsOfInertia=[-5.4062904633677868e-09 -1.3111174919527308e-07 6.0713893531177014e-07]  ProductsOfInertiaUnits=kg*mm^2  BasedOnType=Density  Density=1000  DensityUnits=kg/(m^3)  DoExposeReferenceFrame=on  SerializedFrames=<Frames/>  GraphicType=FromGeometry  MarkerShape=Sphere  MarkerSize=10  MarkerSizeUnits=m  GraphicVisPropType=SimpleVisualProperties  GraphicDiffuseColor=[0.75294117647058822 0.75294117647058822 0.75294117647058822]  GraphicSpecularColor=[0.5 0.5 0.5 1.0]  GraphicAmbientColor=[0.15 0.15 0.15 1.0]  GraphicEmissiveColor=[0.0 0.0 0.0 1.0]  GraphicShininess=75  GraphicOpacity=1  GeometryShape=FromFile  RectangleSize=[1 1]  RectangleSizeUnits=m  BrickDimensions=[1 1 1]  BrickDimensionUnits=m  CylinderRadius=1  CylinderRadiusUnits=m  CylinderLength=1  CylinderLengthUnits=m  SphereRadius=1  SphereRadiusUnits=m  EllipsoidRadii=[1 1 1]  EllipsoidRadiiUnits=m  ExtrusionCrossSection=[1 1; -1 1; -1 -1; 1 -1]  ExtrusionCrossSectionUnits=m  ExtrusionLength=1  ExtrusionLengthUnits=m  PolygonNumSides=3  PolygonOuterRadius=1  PolygonOuterRadiusUnits=m  ExtGeomFileType=STL  ExtGeomFileName=\STL\Vis à tôle tête cylindrique cruciforme H 2-9x13 - C_Réaliste_sldprt.STL  ExtGeomFileUnits=mm  RevolutionCrossSection=[1 1; 1 -1; 2 -1; 2 1]  RevolutionCrossSectionUnits=m  RevolutionExtent=Full  RevolutionAngle=180  RevolutionAngleUnits=deg
  F : PMIOPort  Side=Left
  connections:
  Solid/RConn1 -- ReferenceFrame/RConn1 -- F/RConn1

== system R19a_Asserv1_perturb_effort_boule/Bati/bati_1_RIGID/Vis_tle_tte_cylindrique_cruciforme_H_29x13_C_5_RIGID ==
  ReferenceFrame : sm_lib/Frames and Transforms/Reference Frame
  Solid : sm_lib/Body Elements/Solid  InertiaType=Custom  Mass=8.3821869835456372e-05  MassUnits=kg  CenterOfMass=[4.9478681581074904 0.00064910481891303923 -0.0013634218224953438]  CenterOfMassUnits=mm  MomentsOfInertia=[0.00016543197172893975 0.0014334630955093895 0.0014333390308476422]  MomentsOfInertiaUnits=kg*mm^2  ProductsOfInertia=[-5.4062904633677868e-09 -1.3111174919527308e-07 6.0713893531177014e-07]  ProductsOfInertiaUnits=kg*mm^2  BasedOnType=Density  Density=1000  DensityUnits=kg/(m^3)  DoExposeReferenceFrame=on  SerializedFrames=<Frames/>  GraphicType=FromGeometry  MarkerShape=Sphere  MarkerSize=10  MarkerSizeUnits=m  GraphicVisPropType=SimpleVisualProperties  GraphicDiffuseColor=[0.75294117647058822 0.75294117647058822 0.75294117647058822]  GraphicSpecularColor=[0.5 0.5 0.5 1.0]  GraphicAmbientColor=[0.15 0.15 0.15 1.0]  GraphicEmissiveColor=[0.0 0.0 0.0 1.0]  GraphicShininess=75  GraphicOpacity=1  GeometryShape=FromFile  RectangleSize=[1 1]  RectangleSizeUnits=m  BrickDimensions=[1 1 1]  BrickDimensionUnits=m  CylinderRadius=1  CylinderRadiusUnits=m  CylinderLength=1  CylinderLengthUnits=m  SphereRadius=1  SphereRadiusUnits=m  EllipsoidRadii=[1 1 1]  EllipsoidRadiiUnits=m  ExtrusionCrossSection=[1 1; -1 1; -1 -1; 1 -1]  ExtrusionCrossSectionUnits=m  ExtrusionLength=1  ExtrusionLengthUnits=m  PolygonNumSides=3  PolygonOuterRadius=1  PolygonOuterRadiusUnits=m  ExtGeomFileType=STL  ExtGeomFileName=\STL\Vis à tôle tête cylindrique cruciforme H 2-9x13 - C_Réaliste_sldprt.STL  ExtGeomFileUnits=mm  RevolutionCrossSection=[1 1; 1 -1; 2 -1; 2 1]  RevolutionCrossSectionUnits=m  RevolutionExtent=Full  RevolutionAngle=180  RevolutionAngleUnits=deg
  F : PMIOPort  Side=Left
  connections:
  Solid/RConn1 -- ReferenceFrame/RConn1 -- F/RConn1

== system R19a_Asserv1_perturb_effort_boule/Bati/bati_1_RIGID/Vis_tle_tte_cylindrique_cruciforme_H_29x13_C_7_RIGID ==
  ReferenceFrame : sm_lib/Frames and Transforms/Reference Frame
  Solid : sm_lib/Body Elements/Solid  InertiaType=Custom  Mass=8.3821869835456372e-05  MassUnits=kg  CenterOfMass=[4.9478681581074904 0.00064910481891303923 -0.0013634218224953438]  CenterOfMassUnits=mm  MomentsOfInertia=[0.00016543197172893975 0.0014334630955093895 0.0014333390308476422]  MomentsOfInertiaUnits=kg*mm^2  ProductsOfInertia=[-5.4062904633677868e-09 -1.3111174919527308e-07 6.0713893531177014e-07]  ProductsOfInertiaUnits=kg*mm^2  BasedOnType=Density  Density=1000  DensityUnits=kg/(m^3)  DoExposeReferenceFrame=on  SerializedFrames=<Frames/>  GraphicType=FromGeometry  MarkerShape=Sphere  MarkerSize=10  MarkerSizeUnits=m  GraphicVisPropType=SimpleVisualProperties  GraphicDiffuseColor=[0.75294117647058822 0.75294117647058822 0.75294117647058822]  GraphicSpecularColor=[0.5 0.5 0.5 1.0]  GraphicAmbientColor=[0.15 0.15 0.15 1.0]  GraphicEmissiveColor=[0.0 0.0 0.0 1.0]  GraphicShininess=75  GraphicOpacity=1  GeometryShape=FromFile  RectangleSize=[1 1]  RectangleSizeUnits=m  BrickDimensions=[1 1 1]  BrickDimensionUnits=m  CylinderRadius=1  CylinderRadiusUnits=m  CylinderLength=1  CylinderLengthUnits=m  SphereRadius=1  SphereRadiusUnits=m  EllipsoidRadii=[1 1 1]  EllipsoidRadiiUnits=m  ExtrusionCrossSection=[1 1; -1 1; -1 -1; 1 -1]  ExtrusionCrossSectionUnits=m  ExtrusionLength=1  ExtrusionLengthUnits=m  PolygonNumSides=3  PolygonOuterRadius=1  PolygonOuterRadiusUnits=m  ExtGeomFileType=STL  ExtGeomFileName=\STL\Vis à tôle tête cylindrique cruciforme H 2-9x13 - C_Réaliste_sldprt.STL  ExtGeomFileUnits=mm  RevolutionCrossSection=[1 1; 1 -1; 2 -1; 2 1]  RevolutionCrossSectionUnits=m  RevolutionExtent=Full  RevolutionAngle=180  RevolutionAngleUnits=deg
  F : PMIOPort  Side=Left
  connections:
  Solid/RConn1 -- ReferenceFrame/RConn1 -- F/RConn1

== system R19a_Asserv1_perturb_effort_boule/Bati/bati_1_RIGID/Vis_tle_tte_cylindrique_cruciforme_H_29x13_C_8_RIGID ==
  ReferenceFrame : sm_lib/Frames and Transforms/Reference Frame
  Solid : sm_lib/Body Elements/Solid  InertiaType=Custom  Mass=8.3821869835456372e-05  MassUnits=kg  CenterOfMass=[4.9478681581074904 0.00064910481891303923 -0.0013634218224953438]  CenterOfMassUnits=mm  MomentsOfInertia=[0.00016543197172893975 0.0014334630955093895 0.0014333390308476422]  MomentsOfInertiaUnits=kg*mm^2  ProductsOfInertia=[-5.4062904633677868e-09 -1.3111174919527308e-07 6.0713893531177014e-07]  ProductsOfInertiaUnits=kg*mm^2  BasedOnType=Density  Density=1000  DensityUnits=kg/(m^3)  DoExposeReferenceFrame=on  SerializedFrames=<Frames/>  GraphicType=FromGeometry  MarkerShape=Sphere  MarkerSize=10  MarkerSizeUnits=m  GraphicVisPropType=SimpleVisualProperties  GraphicDiffuseColor=[0.75294117647058822 0.75294117647058822 0.75294117647058822]  GraphicSpecularColor=[0.5 0.5 0.5 1.0]  GraphicAmbientColor=[0.15 0.15 0.15 1.0]  GraphicEmissiveColor=[0.0 0.0 0.0 1.0]  GraphicShininess=75  GraphicOpacity=1  GeometryShape=FromFile  RectangleSize=[1 1]  RectangleSizeUnits=m  BrickDimensions=[1 1 1]  BrickDimensionUnits=m  CylinderRadius=1  CylinderRadiusUnits=m  CylinderLength=1  CylinderLengthUnits=m  SphereRadius=1  SphereRadiusUnits=m  EllipsoidRadii=[1 1 1]  EllipsoidRadiiUnits=m  ExtrusionCrossSection=[1 1; -1 1; -1 -1; 1 -1]  ExtrusionCrossSectionUnits=m  ExtrusionLength=1  ExtrusionLengthUnits=m  PolygonNumSides=3  PolygonOuterRadius=1  PolygonOuterRadiusUnits=m  ExtGeomFileType=STL  ExtGeomFileName=\STL\Vis à tôle tête cylindrique cruciforme H 2-9x13 - C_Réaliste_sldprt.STL  ExtGeomFileUnits=mm  RevolutionCrossSection=[1 1; 1 -1; 2 -1; 2 1]  RevolutionCrossSectionUnits=m  RevolutionExtent=Full  RevolutionAngle=180  RevolutionAngleUnits=deg
  F : PMIOPort  Side=Left
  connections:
  Solid/RConn1 -- ReferenceFrame/RConn1 -- F/RConn1

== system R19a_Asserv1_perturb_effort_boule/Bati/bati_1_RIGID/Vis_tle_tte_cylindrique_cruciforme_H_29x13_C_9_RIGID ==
  ReferenceFrame : sm_lib/Frames and Transforms/Reference Frame
  Solid : sm_lib/Body Elements/Solid  InertiaType=Custom  Mass=8.3821869835456372e-05  MassUnits=kg  CenterOfMass=[4.9478681581074904 0.00064910481891303923 -0.0013634218224953438]  CenterOfMassUnits=mm  MomentsOfInertia=[0.00016543197172893975 0.0014334630955093895 0.0014333390308476422]  MomentsOfInertiaUnits=kg*mm^2  ProductsOfInertia=[-5.4062904633677868e-09 -1.3111174919527308e-07 6.0713893531177014e-07]  ProductsOfInertiaUnits=kg*mm^2  BasedOnType=Density  Density=1000  DensityUnits=kg/(m^3)  DoExposeReferenceFrame=on  SerializedFrames=<Frames/>  GraphicType=FromGeometry  MarkerShape=Sphere  MarkerSize=10  MarkerSizeUnits=m  GraphicVisPropType=SimpleVisualProperties  GraphicDiffuseColor=[0.75294117647058822 0.75294117647058822 0.75294117647058822]  GraphicSpecularColor=[0.5 0.5 0.5 1.0]  GraphicAmbientColor=[0.15 0.15 0.15 1.0]  GraphicEmissiveColor=[0.0 0.0 0.0 1.0]  GraphicShininess=75  GraphicOpacity=1  GeometryShape=FromFile  RectangleSize=[1 1]  RectangleSizeUnits=m  BrickDimensions=[1 1 1]  BrickDimensionUnits=m  CylinderRadius=1  CylinderRadiusUnits=m  CylinderLength=1  CylinderLengthUnits=m  SphereRadius=1  SphereRadiusUnits=m  EllipsoidRadii=[1 1 1]  EllipsoidRadiiUnits=m  ExtrusionCrossSection=[1 1; -1 1; -1 -1; 1 -1]  ExtrusionCrossSectionUnits=m  ExtrusionLength=1  ExtrusionLengthUnits=m  PolygonNumSides=3  PolygonOuterRadius=1  PolygonOuterRadiusUnits=m  ExtGeomFileType=STL  ExtGeomFileName=\STL\Vis à tôle tête cylindrique cruciforme H 2-9x13 - C_Réaliste_sldprt.STL  ExtGeomFileUnits=mm  RevolutionCrossSection=[1 1; 1 -1; 2 -1; 2 1]  RevolutionCrossSectionUnits=m  RevolutionExtent=Full  RevolutionAngle=180  RevolutionAngleUnits=deg
  F : PMIOPort  Side=Left
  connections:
  Solid/RConn1 -- ReferenceFrame/RConn1 -- F/RConn1

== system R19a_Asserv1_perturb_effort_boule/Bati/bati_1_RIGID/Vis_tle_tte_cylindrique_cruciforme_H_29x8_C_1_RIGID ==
  ReferenceFrame : sm_lib/Frames and Transforms/Reference Frame
  Solid : sm_lib/Body Elements/Solid  InertiaType=Custom  Mass=6.1032951855347168e-05  MassUnits=kg  CenterOfMass=[2.8733410905856731 0.00094398948887705679 -0.0019024155537156445]  CenterOfMassUnits=mm  MomentsOfInertia=[0.0001480040782382925 0.00040137501597657324 0.00040131942245693811]  MomentsOfInertiaUnits=kg*mm^2  ProductsOfInertia=[3.5650623197794874e-09 -1.4668534891118034e-08 2.7820926592949074e-07]  ProductsOfInertiaUnits=kg*mm^2  BasedOnType=Density  Density=1000  DensityUnits=kg/(m^3)  DoExposeReferenceFrame=on  SerializedFrames=<Frames/>  GraphicType=FromGeometry  MarkerShape=Sphere  MarkerSize=10  MarkerSizeUnits=m  GraphicVisPropType=SimpleVisualProperties  GraphicDiffuseColor=[0.75294117647058822 0.75294117647058822 0.75294117647058822]  GraphicSpecularColor=[0.5 0.5 0.5 1.0]  GraphicAmbientColor=[0.15 0.15 0.15 1.0]  GraphicEmissiveColor=[0.0 0.0 0.0 1.0]  GraphicShininess=75  GraphicOpacity=1  GeometryShape=FromFile  RectangleSize=[1 1]  RectangleSizeUnits=m  BrickDimensions=[1 1 1]  BrickDimensionUnits=m  CylinderRadius=1  CylinderRadiusUnits=m  CylinderLength=1  CylinderLengthUnits=m  SphereRadius=1  SphereRadiusUnits=m  EllipsoidRadii=[1 1 1]  EllipsoidRadiiUnits=m  ExtrusionCrossSection=[1 1; -1 1; -1 -1; 1 -1]  ExtrusionCrossSectionUnits=m  ExtrusionLength=1  ExtrusionLengthUnits=m  PolygonNumSides=3  PolygonOuterRadius=1  PolygonOuterRadiusUnits=m  ExtGeomFileType=STL  ExtGeomFileName=\STL\Vis à tôle tête cylindrique cruciforme H 2-9x8 - C_Réaliste_sldprt.STL  ExtGeomFileUnits=mm  RevolutionCrossSection=[1 1; 1 -1; 2 -1; 2 1]  RevolutionCrossSectionUnits=m  RevolutionExtent=Full  RevolutionAngle=180  RevolutionAngleUnits=deg
  F : PMIOPort  Side=Left
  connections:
  Solid/RConn1 -- ReferenceFrame/RConn1 -- F/RConn1

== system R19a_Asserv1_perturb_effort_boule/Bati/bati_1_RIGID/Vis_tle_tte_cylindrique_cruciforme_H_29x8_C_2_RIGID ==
  ReferenceFrame : sm_lib/Frames and Transforms/Reference Frame
  Solid : sm_lib/Body Elements/Solid  InertiaType=Custom  Mass=6.1032951855347168e-05  MassUnits=kg  CenterOfMass=[2.8733410905856731 0.00094398948887705679 -0.0019024155537156445]  CenterOfMassUnits=mm  MomentsOfInertia=[0.0001480040782382925 0.00040137501597657324 0.00040131942245693811]  MomentsOfInertiaUnits=kg*mm^2  ProductsOfInertia=[3.5650623197794874e-09 -1.4668534891118034e-08 2.7820926592949074e-07]  ProductsOfInertiaUnits=kg*mm^2  BasedOnType=Density  Density=1000  DensityUnits=kg/(m^3)  DoExposeReferenceFrame=on  SerializedFrames=<Frames/>  GraphicType=FromGeometry  MarkerShape=Sphere  MarkerSize=10  MarkerSizeUnits=m  GraphicVisPropType=SimpleVisualProperties  GraphicDiffuseColor=[0.75294117647058822 0.75294117647058822 0.75294117647058822]  GraphicSpecularColor=[0.5 0.5 0.5 1.0]  GraphicAmbientColor=[0.15 0.15 0.15 1.0]  GraphicEmissiveColor=[0.0 0.0 0.0 1.0]  GraphicShininess=75  GraphicOpacity=1  GeometryShape=FromFile  RectangleSize=[1 1]  RectangleSizeUnits=m  BrickDimensions=[1 1 1]  BrickDimensionUnits=m  CylinderRadius=1  CylinderRadiusUnits=m  CylinderLength=1  CylinderLengthUnits=m  SphereRadius=1  SphereRadiusUnits=m  EllipsoidRadii=[1 1 1]  EllipsoidRadiiUnits=m  ExtrusionCrossSection=[1 1; -1 1; -1 -1; 1 -1]  ExtrusionCrossSectionUnits=m  ExtrusionLength=1  ExtrusionLengthUnits=m  PolygonNumSides=3  PolygonOuterRadius=1  PolygonOuterRadiusUnits=m  ExtGeomFileType=STL  ExtGeomFileName=\STL\Vis à tôle tête cylindrique cruciforme H 2-9x8 - C_Réaliste_sldprt.STL  ExtGeomFileUnits=mm  RevolutionCrossSection=[1 1; 1 -1; 2 -1; 2 1]  RevolutionCrossSectionUnits=m  RevolutionExtent=Full  RevolutionAngle=180  RevolutionAngleUnits=deg
  F : PMIOPort  Side=Left
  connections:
  Solid/RConn1 -- ReferenceFrame/RConn1 -- F/RConn1

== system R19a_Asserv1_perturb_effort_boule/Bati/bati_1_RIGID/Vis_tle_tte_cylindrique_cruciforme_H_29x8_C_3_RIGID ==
  ReferenceFrame : sm_lib/Frames and Transforms/Reference Frame
  Solid : sm_lib/Body Elements/Solid  InertiaType=Custom  Mass=6.1032951855347168e-05  MassUnits=kg  CenterOfMass=[2.8733410905856731 0.00094398948887705679 -0.0019024155537156445]  CenterOfMassUnits=mm  MomentsOfInertia=[0.0001480040782382925 0.00040137501597657324 0.00040131942245693811]  MomentsOfInertiaUnits=kg*mm^2  ProductsOfInertia=[3.5650623197794874e-09 -1.4668534891118034e-08 2.7820926592949074e-07]  ProductsOfInertiaUnits=kg*mm^2  BasedOnType=Density  Density=1000  DensityUnits=kg/(m^3)  DoExposeReferenceFrame=on  SerializedFrames=<Frames/>  GraphicType=FromGeometry  MarkerShape=Sphere  MarkerSize=10  MarkerSizeUnits=m  GraphicVisPropType=SimpleVisualProperties  GraphicDiffuseColor=[0.75294117647058822 0.75294117647058822 0.75294117647058822]  GraphicSpecularColor=[0.5 0.5 0.5 1.0]  GraphicAmbientColor=[0.15 0.15 0.15 1.0]  GraphicEmissiveColor=[0.0 0.0 0.0 1.0]  GraphicShininess=75  GraphicOpacity=1  GeometryShape=FromFile  RectangleSize=[1 1]  RectangleSizeUnits=m  BrickDimensions=[1 1 1]  BrickDimensionUnits=m  CylinderRadius=1  CylinderRadiusUnits=m  CylinderLength=1  CylinderLengthUnits=m  SphereRadius=1  SphereRadiusUnits=m  EllipsoidRadii=[1 1 1]  EllipsoidRadiiUnits=m  ExtrusionCrossSection=[1 1; -1 1; -1 -1; 1 -1]  ExtrusionCrossSectionUnits=m  ExtrusionLength=1  ExtrusionLengthUnits=m  PolygonNumSides=3  PolygonOuterRadius=1  PolygonOuterRadiusUnits=m  ExtGeomFileType=STL  ExtGeomFileName=\STL\Vis à tôle tête cylindrique cruciforme H 2-9x8 - C_Réaliste_sldprt.STL  ExtGeomFileUnits=mm  RevolutionCrossSection=[1 1; 1 -1; 2 -1; 2 1]  RevolutionCrossSectionUnits=m  RevolutionExtent=Full  RevolutionAngle=180  RevolutionAngleUnits=deg
  F : PMIOPort  Side=Left
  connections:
  Solid/RConn1 -- ReferenceFrame/RConn1 -- F/RConn1
